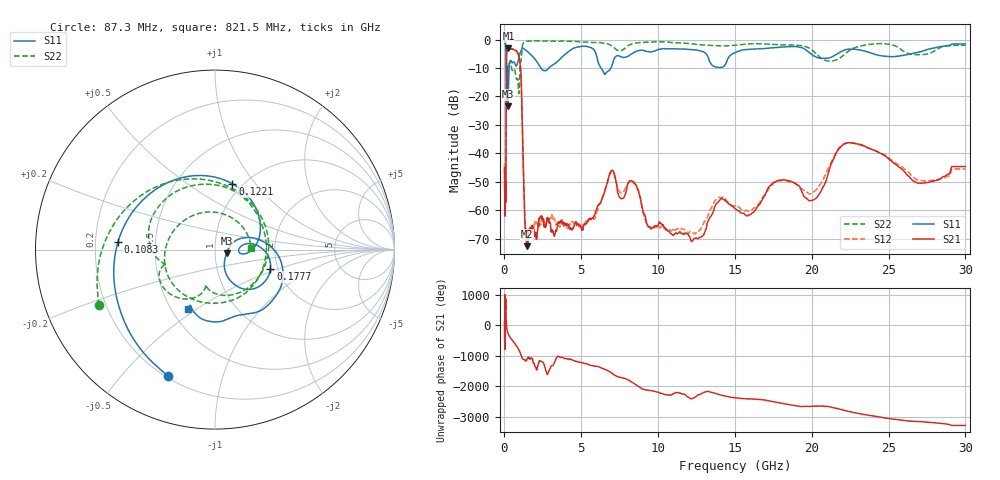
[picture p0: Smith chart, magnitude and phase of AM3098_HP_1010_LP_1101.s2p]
! Date/Time: Thu, Feb 28, 2019 8:42 AM
! Network Analyzer: Agilent Technologies E8364B Rev: A.07.50.67
! Sweep from 0.010 to 30.000 GHz, 1601 Points, Sweep Type: LOG
! Power Supply: 5.023 V, 0.002 A
# Hz S DB R 50
!freq MagS11 AngS11 MagS21 AngS21 MagS12 AngS12 MagS22 AngS22
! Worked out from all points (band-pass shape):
!   1601 points, 10 MHz to 30 GHz, reference 50 ohm
!   highest |S21| = -3.12 dB at 258.6 MHz (marker M1); lowest = -72.7 dB at 1.453 GHz (marker M2)
!   |S21| within 3 dB of the highest: 133.8 MHz to 944.1 MHz (810.2 MHz wide, 150 % of centre)
!   lowest |S11| = -23.4 dB at 241.1 MHz (marker M3), VSWR 1.14, Z = 56.8 - j2.33 ohm
!   |S11| at or under -10 dB: 192.8 MHz to 301.6 MHz (108.8 MHz wide, 44 % of centre); 2.37 GHz to 2.901 GHz (530.9 MHz wide, 20.1 % of centre); 6.284 GHz to 6.935 GHz (650.7 MHz wide, 9.84 % of centre)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
!   |S22| runs from -19.0 to -0.4 dB; largest |S21 - S12| = 0.011
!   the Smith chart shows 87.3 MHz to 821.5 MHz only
!   S11 on the Smith chart (normalised r, x): 87.3 MHz: 0.21, -0.67; 108.3 MHz: 0.30, +0.04; 122.1 MHz: 0.90, +0.77; 177.7 MHz: 1.82, -0.44; 821.5 MHz: 0.61, -0.46
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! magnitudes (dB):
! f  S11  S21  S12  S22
! 10 MHz  -0.3  -46.8  -44.4  -0.6
! 38.04 MHz  -0.4  -60.1  -58.0  -1.0
! 87.3 MHz  -2.5  -54.5  -54.3  -2.9
! 108.3 MHz  -5.3  -30.4  -30.4  -6.8
! 122.1 MHz  -8.4  -12.2  -12.2  -10.6
! 144.7 MHz  -17.6  -4.7  -4.7  -13.7
! 177.7 MHz  -9.7  -3.8  -3.8  -9.1
! 241.1 MHz  -23.4  -3.1  -3.1  -11.0
! 258.6 MHz  -17.9  -3.1  -3.1  -10.6
! 550.5 MHz  -8.1  -3.5  -3.4  -10.7
! 821.5 MHz  -8.8  -4.3  -4.3  -13.9
! 1.066 GHz  -4.3  -11.4  -11.4  -7.8
! 1.321 GHz  -3.5  -62.9  -63.6  -0.8
! 1.453 GHz  -4.0  -72.7  -67.6  -0.6
! 2.084 GHz  -7.6  -70.2  -64.0  -0.4
! 5.002 GHz  -2.4  -66.3  -66.3  -0.8
! 6.924 GHz  -10.1  -46.3  -46.7  -2.0
! 7.926 GHz  -6.2  -53.2  -51.5  -2.7
! 12.5 GHz  -3.7  -69.8  -67.9  -1.7
! 20.1 GHz  -5.6  -56.4  -53.7  -4.1
! 22.56 GHz  -3.4  -36.3  -36.3  -3.5
! 30 GHz  -1.6  -44.7  -45.5  -2.0
